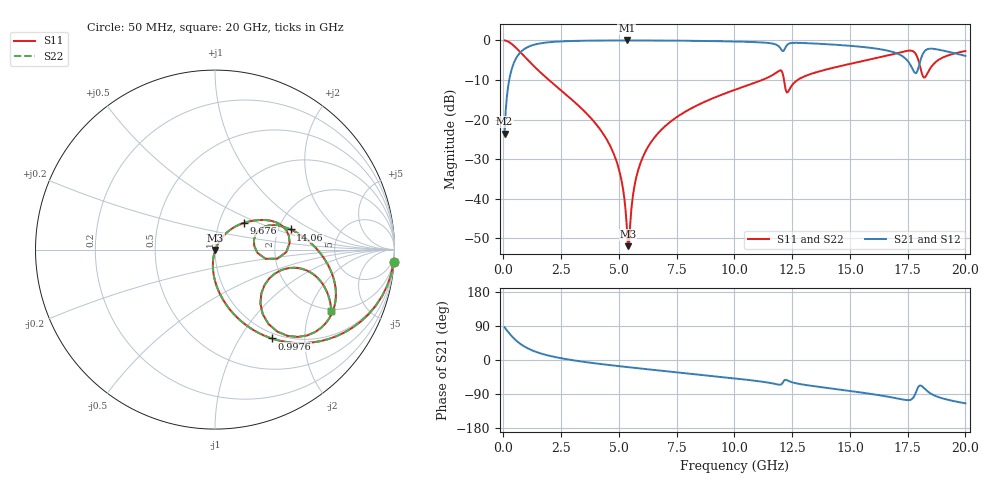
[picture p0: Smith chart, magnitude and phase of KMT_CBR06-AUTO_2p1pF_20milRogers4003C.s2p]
! Data measured by Modelithics Inc. support@modelithics.com 813-866-6335
! KEMET CBR06-AUTO 2.1pF, Pad Width= 0.851mm, Pad Length= 0.64mm, Pad Gap= 0.62mm, 20mil Rogers 4003C substrate Data, January 2022
# hz S ma R 50
! 2 Port Network Data from SP1.SP block
! freq  magS11  angS11  magS21  angS21  magS12  angS12  magS22  angS22
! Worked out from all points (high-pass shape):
!   401 points, 50 MHz to 20 GHz, reference 50 ohm
!   highest |S21| = -0.02 dB at 5.337 GHz (marker M1); lowest = -23.5 dB at 50 MHz (marker M2)
!   |S21| within 3 dB of the highest: 736.1 MHz to 16.91 GHz (16.17 GHz wide, 183 % of centre); 18.2 GHz to 19.37 GHz (1.176 GHz wide, 6.26 % of centre)
!   lowest |S11| = -52.0 dB at 5.387 GHz (marker M3), VSWR 1.01, Z = 50.2 - j0.194 ohm
!   |S11| at or under -10 dB: 1.967 GHz to 11.2 GHz (9.233 GHz wide, 140 % of centre); 12.14 GHz to 12.74 GHz (592 MHz wide, 4.76 % of centre)
!   |S22| runs from -52.0 to 0.0 dB; largest |S21 - S12| = 0
!   S11 on the Smith chart (normalised r, x): 50 MHz: 1, -29; 997.6 MHz: 0.92, -1.39; 9.676 GHz: 1.31, +0.41; 14.06 GHz: 2.33, +0.64; 20 GHz: 1.92, -2.84
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5e7  0.9978 -4.0  0.06665 86.0  0.06665 86.0  0.9978 -4.0
3.99125e8  0.881 -29.6  0.4721 60.4  0.4721 60.4  0.881 -29.6
9.97625e8  0.5874 -57.4  0.808 32.4  0.808 32.4  0.5874 -57.4
3.391625e9  0.1369 -93.3  0.9886 -4.1  0.9886 -4.1  0.1369 -93.3
4.788125e9  0.03614 -101.5  0.9971 -14.8  0.9971 -14.8  0.03614 -101.5
5.13725e9  0.01556 -99.4  0.9976 -17.2  0.9976 -17.2  0.01556 -99.4
5.33675e9  0.004621 -80.9  0.9977 -18.5  0.9977 -18.5  0.004621 -80.9
5.386625e9  0.002519 -50.1  0.9977 -18.9  0.9977 -18.9  0.002519 -50.1
5.885375e9  0.02578 62.9  0.9972 -22.1  0.9972 -22.1  0.02578 62.9
6.73325e9  0.06917 60.5  0.995 -27.6  0.995 -27.6  0.06917 60.5
9.675875e9  0.2183 42.9  0.9723 -46.3  0.9723 -46.3  0.2183 42.9
1.0025e10  0.2378 40.5  0.9674 -48.6  0.9674 -48.6  0.2378 40.5
1.192025e10  0.4123 14.8  0.8414 -65.2  0.8414 -65.2  0.4123 14.8
1.216962e10  0.2861 -10.2  0.7713 -53.3  0.7713 -53.3  0.2861 -10.2
1.336662e10  0.3814 20.3  0.9156 -68.4  0.9156 -68.4  0.3814 20.3
1.406488e10  0.4354 14.9  0.8925 -74.1  0.8925 -74.1  0.4354 14.9
1.670825e10  0.6507 -9.7  0.7333 -97.4  0.7333 -97.4  0.6507 -9.7
1.755612e10  0.7422 -28.8  0.5243 -105.9  0.5243 -105.9  0.7422 -28.8
1.785538e10  0.6707 -46.5  0.3844 -85.5  0.3844 -85.5  0.6707 -46.5
1.810475e10  0.3922 -49.9  0.6198 -68.5  0.6198 -68.5  0.3922 -49.9
1.850375e10  0.4543 -12.9  0.786 -88.7  0.786 -88.7  0.4543 -12.9
2e10  0.733 -27.8  0.6359 -114.3  0.6359 -114.3  0.733 -27.8
